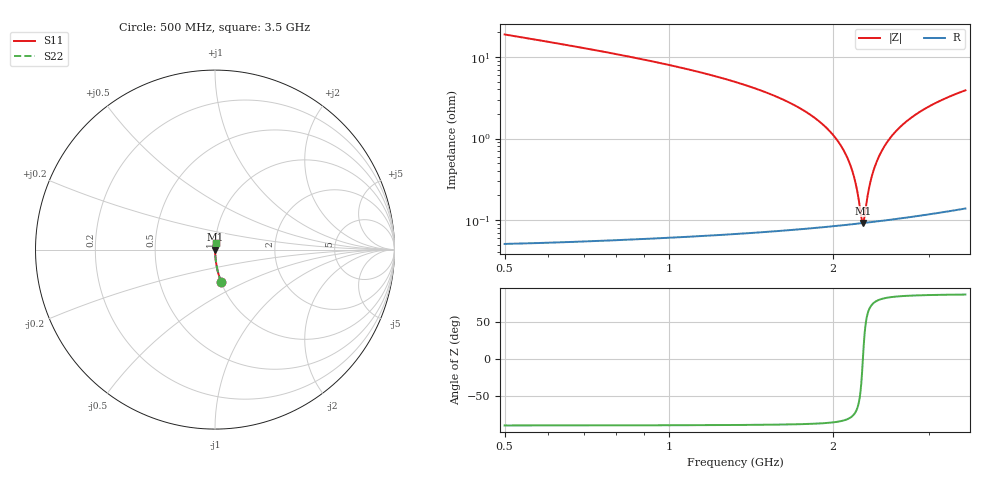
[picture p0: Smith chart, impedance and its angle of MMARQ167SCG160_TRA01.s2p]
! MMARQ167SCG160_TRA01  S-PARAMETER MODEL  ( General Type )
! Model Generated by TAIYO YUDEN Corporation (http://www.ty-top.com)
! Version 1.0
! TAIYO YUDEN Control No. 160201
! Copyright(c) 2016 TAIYO YUDEN CO.,LTD. All Rights Reserved.
! Product Description (link to TY-COMPAS)
! https://ds.yuden.co.jp/TYCOMPAS/or/detail?pn=MMARQ167SCG160JTRA01&u=M
! Products Name : Multilayer Ceramic Capacitors
! Characteristics :
!  Capacitance : 16 pF , Rated Voltage : 250V , TCC : CG / C0G
!  Case Size : 1.6 x 0.8 / 0.063 x 0.031 [mm/inch] , Thickness : 0.7 / 0.028 [mm/inch]
!  (Conditions: Temperature = 25 degC , DC Bias Current/Voltage = 0A / 0V)
! External Node Assignments :
!  1  o---| |---o  2
! GND o---------o GND
! Frequency Range : 500MHz  -  3500MHz  [ 401 STEP ]
# MHz S RI R 50
! Freq[MHz].  S11 Real  S11 Imag  S21 Real  S21 Imag  S12 Real  S12 Imag  S22 Real  S22 Imag
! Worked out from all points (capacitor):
!   401 points, 500 MHz to 3.5 GHz, reference 50 ohm
!   read as one part in series: C = 16 pF near 515 MHz
!   lowest |Z| = 91.7 mohm at 2.27 GHz (marker M1)
!   series resonance near 2.27 GHz, so ESL is about 310 pH
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500  0.035 -0.1824  0.965 0.1824  0.965 0.1824  0.035 -0.1824
725  0.0154 -0.1211  0.9846 0.1211  0.9846 0.1211  0.0154 -0.1211
1002.5  0.00692 -0.0792  0.9931 0.0792  0.9931 0.0792  0.00692 -0.0792
1505  0.00208 -0.0369  0.9979 0.0369  0.9979 0.0369  0.00208 -0.0369
1797.5  0.00121 -0.0206  0.9988 0.0206  0.9988 0.0206  0.00121 -0.0206
1910  0.00104 -0.0152  0.999 0.0152  0.999 0.0152  0.00104 -0.0152
2000  0.00096 -0.0111  0.999 0.0111  0.999 0.0111  0.00096 -0.0111
2090  0.000915 -0.00722  0.9991 0.00722  0.9991 0.00722  0.000915 -0.00722
2157.5  0.000902 -0.00444  0.9991 0.00444  0.9991 0.00444  0.000902 -0.00444
2202.5  0.000903 -0.00264  0.9991 0.00264  0.9991 0.00264  0.000903 -0.00264
2225  0.000906 -0.00175  0.9991 0.00175  0.9991 0.00175  0.000906 -0.00175
2255  0.000912 -0.00058  0.9991 0.00058  0.9991 0.00058  0.000912 -0.00058
2270  0.000916 -1.45e-06  0.9991 1.45e-06  0.9991 1.45e-06  0.000916 -1.45e-06
2285  0.000921 0.000573  0.9991 -0.000573  0.9991 -0.000573  0.000921 0.000573
2330  0.00094 0.00228  0.9991 -0.00228  0.9991 -0.00228  0.00094 0.00228
2367.5  0.00096 0.00367  0.999 -0.00367  0.999 -0.00367  0.00096 0.00367
2427.5  0.001 0.00586  0.999 -0.00586  0.999 -0.00586  0.001 0.00586
2502.5  0.00106 0.00852  0.9989 -0.00852  0.9989 -0.00852  0.00106 0.00852
2592.5  0.00116 0.0116  0.9988 -0.0116  0.9988 -0.0116  0.00116 0.0116
2705  0.0013 0.0154  0.9987 -0.0154  0.9987 -0.0154  0.0013 0.0154
3005  0.00179 0.0248  0.9982 -0.0248  0.9982 -0.0248  0.00179 0.0248
3500  0.00289 0.0389  0.9971 -0.0389  0.9971 -0.0389  0.00289 0.0389
